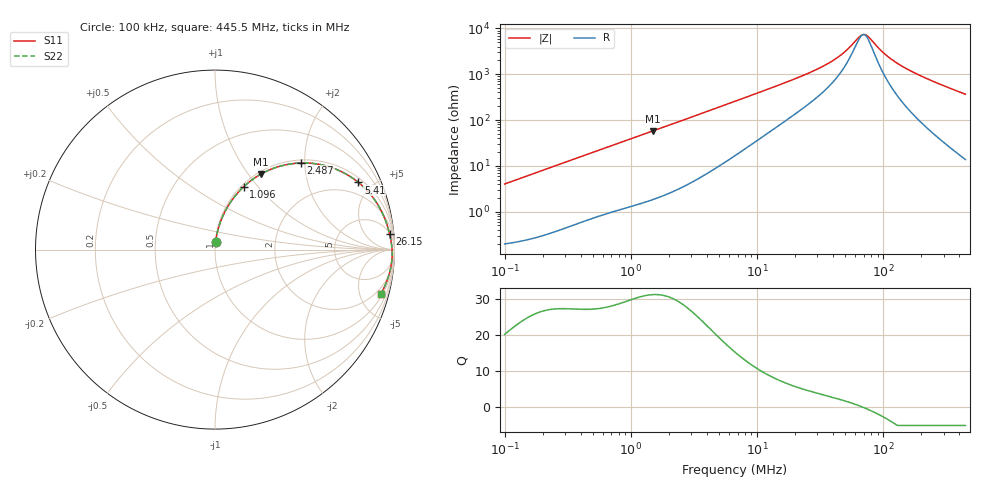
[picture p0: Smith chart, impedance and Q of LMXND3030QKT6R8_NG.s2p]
! LMXND3030QKT6R8_NG  S-PARAMETER MODEL  ( General Type )
! Model Generated by TAIYO YUDEN Corporation (https://www.yuden.co.jp/en/)
! Version 1.0
! TAIYO YUDEN Control No. 191023NI43SB-FBB
! Copyright(c) 2019 TAIYO YUDEN CO.,LTD. All Rights Reserved.
! Product Description (link to TY-COMPAS)
! https://ds.yuden.co.jp/TYCOMPAS/or/detail?pn=LMXND3030QKT6R8MNG&u=M
! Products Name : Inductors
! Characteristics :
!  Inductance : 6.8 uH , SRF(min) : 36 MHz , DC Resistance(max) : 0.192 Ohm
!  Rated Current : Saturation :870 mA , Temp Rise : 880 mA (40 degC)
!  Case Size : 3.0 x 3.0 / 0.118 x 0.118 [mm/inch] , Thickness : 1.5 / 0.059 [mm/inch]
!  (Conditions: Temperature = 25 degC , DC Bias Current/Voltage = 0A / 0V)
! External Node Assignments :
!  1  o---GGG---o  2
! GND o---------o GND
! Frequency Range : 0.1MHz  -  445.549718MHz  [ 402 STEP ]
# MHz S RI R 50
! Freq[MHz].  S11 Real  S11 Imag  S21 Real  S21 Imag  S12 Real  S12 Imag  S22 Real  S22 Imag
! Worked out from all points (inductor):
!   401 points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, 100 kHz to 445.5 MHz, reference 50 ohm
!   read as one part in series: L = 6.38 uH near 104.3 kHz
!   highest Q = 31.3 at 1.502 MHz (marker M1), where L = 6.13 uH
!   self-resonance near 69.35 MHz
!   S11 on the Smith chart (normalised r, x): 100 kHz: 1.00, +0.08; 1.096 MHz: 1.03, +0.85; 2.487 MHz: 1.07, +1.91; 5.41 MHz: 1.23, +4.15; 26.15 MHz: 6, +21; 445.5 MHz: 1.27, -7.32
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0.1  0.00358 0.0399  0.9964 -0.0399  0.9964 -0.0399  0.00358 0.0399
0.408498  0.0308 0.1555  0.9692 -0.1555  0.9692 -0.1555  0.0308 0.1555
0.705291  0.0781 0.2512  0.9219 -0.2512  0.9219 -0.2512  0.0781 0.2512
1.096315  0.1606 0.3511  0.8394 -0.3511  0.8394 -0.3511  0.1606 0.3511
1.502343  0.2579 0.4218  0.7421 -0.4218  0.7421 -0.4218  0.2579 0.4218
1.668708  0.2982 0.4418  0.7018 -0.4418  0.7018 -0.4418  0.2982 0.4418
2.487155  0.4782 0.4826  0.5218 -0.4826  0.5218 -0.4826  0.4782 0.4826
3.480636  0.6359 0.4614  0.3641 -0.4614  0.3641 -0.4614  0.6359 0.4614
5.410354  0.7993 0.374  0.2007 -0.374  0.2007 -0.374  0.7993 0.374
6.81664  0.8573 0.3182  0.1427 -0.3182  0.1427 -0.3182  0.8573 0.3182
11.76924  0.9347 0.1991  0.0653 -0.1991  0.0653 -0.1991  0.9347 0.1991
26.14531  0.973 0.0856  0.027 -0.0856  0.027 -0.0856  0.973 0.0856
27.26705  0.974 0.0812  0.026 -0.0812  0.026 -0.0812  0.974 0.0812
44.20279  0.9826 0.0368  0.0174 -0.0368  0.0174 -0.0368  0.9826 0.0368
64.51342  0.9862 0.0059  0.0138 -0.0059  0.0138 -0.0059  0.9862 0.0059
68.7095  0.9865 0.000762  0.0135 -0.000762  0.0135 -0.000762  0.9865 0.000762
76.31817  0.987 -0.00789  0.013 0.00789  0.013 0.00789  0.987 -0.00789
94.15652  0.9872 -0.0258  0.0128 0.0258  0.0128 0.0258  0.9872 -0.0258
111.3854  0.9867 -0.0411  0.0133 0.0411  0.0133 0.0411  0.9867 -0.0411
140.3372  0.9848 -0.0642  0.0152 0.0642  0.0152 0.0642  0.9848 -0.0642
192.3121  0.979 -0.1012  0.021 0.1012  0.021 0.1012  0.979 -0.1012
445.5497  0.9226 -0.2491  0.0774 0.2491  0.0774 0.2491  0.9226 -0.2491
